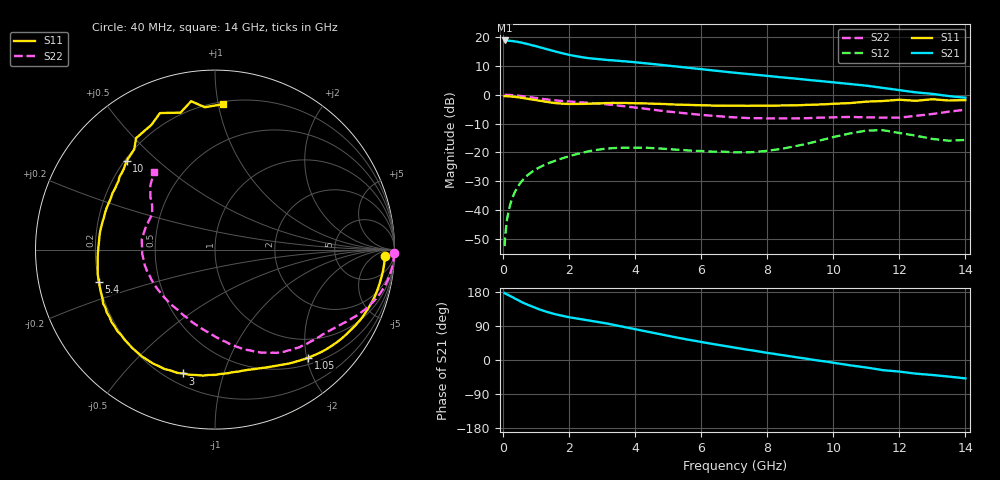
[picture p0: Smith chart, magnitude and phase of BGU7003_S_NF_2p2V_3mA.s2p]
!	Filename:	P:\Prog\Test\Noise\ATS_data\Testdata_Net\BGU7002	BGU7003	RN20082092\BGU7003_B1_high	freq_bias	loop_2.2V2.73mA_D.s2p
!	Date/Time:	Tue	16-Sep-08	9:20:55
!	BGU7003_B1_high	freq_bias	loop
!	bias	mode	1:00	Vout=	2.2	"V,"	Iout=	2.722	"mA,"	Vin=	1.8327	"V,"	Iin=	0.286	mA
!	Date/time	Tue	Aug	12	15:20:33	2008
!	Device	data	file	deembeded	for	feedlines	and	parallel
!	Original	file:	\BGU7002	BGU7003	RN20082092\BGU7003_B1_high	freq_bias	loop_2.2V2.73mA_R.s2p
!	Feed-files:	PR029V01_high	"frequency_140808_Feed1.s2p,"	PR029V01_high	frequency_140808_Feed2.s2p
!	Parallel-file:	PR029V01_high	frequency_140808_Par.s2p
#	MHz	S	MA	R	50
!	Freq-MHz	S11-mag	S11-arg	S21-mag	S21-arg	S12-mag	S12-arg	S22-mag	S22-arg
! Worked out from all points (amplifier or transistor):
!   144 points, 40 MHz to 14 GHz, reference 50 ohm
!   highest |S21| = 18.9 dB at 50 MHz (marker M1)
!   |S21| within 3 dB of that: start of sweep to 1.309 GHz
!   unconditionally stable (mu >= 1): nowhere
!   at 280 MHz: K = 0.09, MSG = 27.2 dB, |S12| = -35.7 dB
!   at 1.85 GHz: K = 0.40, MSG = 18.1 dB, |S12| = -21.8 dB
!   at 14 GHz: K = 0.73, MSG = 7.3 dB, |S12| = -15.7 dB
!   lowest NFmin = 0.42 dB at 400 MHz
!   S11 on the Smith chart (normalised r, x): 40 MHz: 25, -17; 1.05 GHz: 0.62, -2.03; 3 GHz: 0.26, -0.74; 5.4 GHz: 0.20, -0.13; 10 GHz: 0.21, +0.40; 14 GHz: 0.22, +1.03
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40  0.9477 -2.1  8.786 176.6  0.00234 86.9  0.9993 -1.1
50  0.9463 -2.7  8.798 175.9  0.00296 87.7  0.9984 -1.4
120  0.9444 -6.5  8.748 172.9  0.00713 85.9  0.9964 -3.4
210  0.9369 -11.3  8.65 168.9  0.01238 83.2  0.9912 -6.0
410  0.9125 -21.6  8.378 159.7  0.02366 77.2  0.9711 -11.3
550  0.8889 -28.4  8.062 153.1  0.03106 73.2  0.9521 -14.9
750  0.8524 -37.4  7.592 145.4  0.04063 68.1  0.9192 -19.4
1050  0.7954 -49.2  6.84 135.0  0.05306 61.9  0.8699 -25.1
1350  0.7446 -59.4  6.138 126.2  0.06392 57.0  0.8255 -29.7
1650  0.7113 -67.9  5.515 119.3  0.07417 52.9  0.7926 -33.8
2000  0.6919 -77.2  4.939 112.7  0.08575 48.1  0.7624 -38.5
2400  0.6935 -87.5  4.484 107.0  0.09862 42.4  0.7371 -44.3
3000  0.7128 -104.5  4.098 98.3  0.1138 31.9  0.6936 -54.1
3700  0.721 -124.3  3.815 86.6  0.1204 20.8  0.6301 -65.8
4700  0.6975 -149.7  3.348 68.6  0.1171 9.5  0.5346 -80.6
5400  0.672 -164.4  3.034 56.9  0.1104 6.4  0.4834 -90.2
6200  0.6526 -178.5  2.701 44.4  0.1035 5.9  0.4382 -101.9
7200  0.6457 166.6  2.363 30.0  0.1001 9.5  0.4007 -118.5
9400  0.6722 140.6  1.776 0.6  0.1505 21.7  0.3972 -162.7
10000  0.6979 134.8  1.645 -7.2  0.1843 17.7  0.4061 -176.4
12000  0.8201 111.9  1.205 -30.6  0.2168 -24.4  0.4006 150.7
14000  0.8109 87.0  0.8899 -48.5  0.1645 -27.1  0.5504 128.0
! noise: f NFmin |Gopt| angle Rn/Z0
400  0.42  0.51  12.87  0.21
1000  0.56  0.49  27.43  0.21
1500  0.67  0.48  39.56  0.21
1700  0.71  0.48  44.42  0.2
2200  0.83  0.47  56.55  0.19
3000  1.01  0.45  75.96  0.18
4400  1.32  0.45  109.9  0.13
5800  1.64  0.45  143.9  0.1
8000  2.14  0.5  -170.9  0.09
1.2e+04  3.04  0.68  -128.6  0.42
